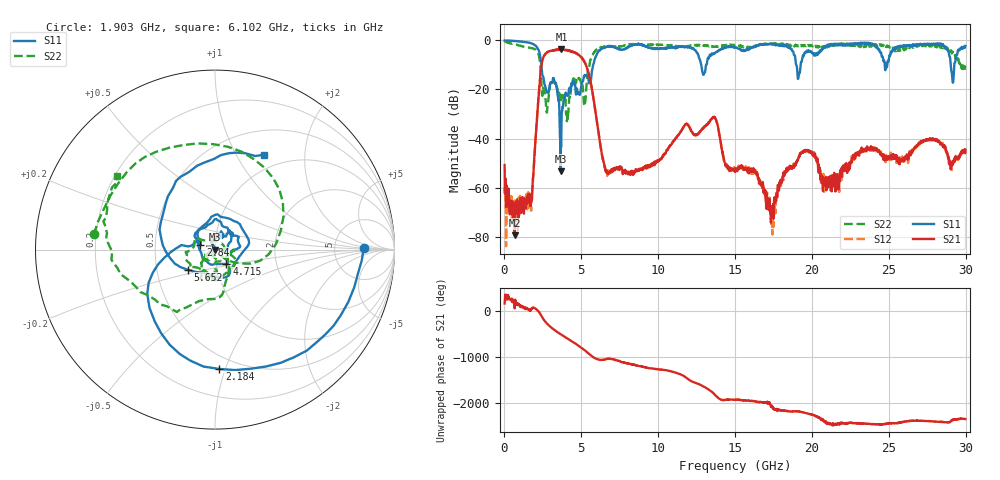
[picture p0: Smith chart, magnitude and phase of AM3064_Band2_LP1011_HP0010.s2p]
# Hz S DB R 50.0
!freq dBS11 angS11 dBS21 angS21 dBS12 angS12 dBS22 angS22
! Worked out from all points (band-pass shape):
!   1600 points, 10 MHz to 29.98 GHz, reference 50 ohm
!   highest |S21| = -3.65 dB at 3.703 GHz (marker M1); lowest = -79.4 dB at 666 MHz (marker M2)
!   |S21| within 3 dB of the highest: 2.547 GHz to 4.955 GHz (2.408 GHz wide, 64.2 % of centre)
!   lowest |S11| = -53.3 dB at 3.646 GHz (marker M3), VSWR 1.00, Z = 49.8 - j0.0542 ohm
!   |S11| at or under -10 dB: 2.396 GHz to 5.772 GHz (3.376 GHz wide, 82.7 % of centre); 12.8 GHz to 13.12 GHz (320.3 MHz wide, 2.47 % of centre); 18.98 GHz to 19.27 GHz (290.1 MHz wide, 1.52 % of centre)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
!   |S22| runs from -33.0 to -0.3 dB; largest |S21 - S12| = 0.022
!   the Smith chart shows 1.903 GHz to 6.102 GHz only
!   S11 on the Smith chart (normalised r, x): 1.903 GHz: 11, +1; 2.184 GHz: 0.40, -0.95; 2.84 GHz: 0.85, +0.05; 4.715 GHz: 1.12, -0.19; 5.652 GHz: 0.72, -0.17; 6.102 GHz: 0.80, +1.31
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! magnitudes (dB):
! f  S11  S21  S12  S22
! 10 MHz  0.0  -50.8  -59.8  -0.3
! 666 MHz  -0.3  -79.4  -65.3  -1.6
! 1.903 GHz  -1.6  -52.1  -51.9  -3.4
! 2.184 GHz  -3.5  -25.9  -25.9  -5.2
! 2.84 GHz  -21.3  -4.6  -4.6  -25.0
! 3.29 GHz  -17.1  -4.0  -4.0  -17.7
! 3.646 GHz  -53.3  -3.7  -3.9  -25.4
! 3.703 GHz  -35.7  -3.6  -3.9  -22.5
! 4.715 GHz  -19.7  -5.5  -5.4  -15.3
! 5.015 GHz  -17.4  -7.1  -6.9  -18.4
! 5.652 GHz  -14.5  -18.4  -18.5  -7.3
! 6.102 GHz  -4.5  -36.9  -36.8  -3.3
! 6.72 GHz  -2.6  -53.7  -52.9  -2.4
! 10 GHz  -3.4  -49.3  -49.0  -1.9
! 13.6 GHz  -5.3  -31.7  -31.4  -2.5
! 15 GHz  -2.6  -53.7  -52.4  -1.9
! 17.42 GHz  -1.6  -70.3  -79.1  -1.5
! 19.99 GHz  -4.6  -45.6  -45.6  -2.0
! 20.85 GHz  -2.8  -58.1  -58.2  -2.6
! 25 GHz  -8.0  -47.4  -48.7  -2.3
! 29.18 GHz  -17.3  -49.9  -49.6  -4.8
! 29.98 GHz  -2.3  -44.7  -45.4  -10.2
